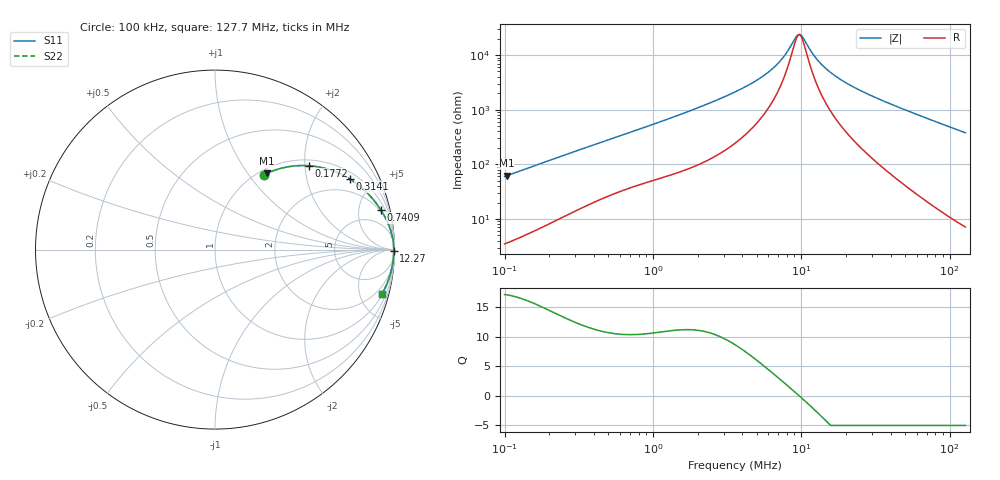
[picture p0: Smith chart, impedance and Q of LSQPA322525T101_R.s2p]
! LSQPA322525T101_R  S-PARAMETER MODEL  ( General Type )
! Model Generated by TAIYO YUDEN Corporation (http://www.ty-top.com)
! Version 2.0
! TAIYO YUDEN Control No. 100810NF25SB-FAC
! Copyright(c) 2007 TAIYO YUDEN CO.,LTD. All Rights Reserved.
! Product Description (link to TY-COMPAS)
! https://ds.yuden.co.jp/TYCOMPAS/or/detail?pn=LSQPA322525T101KR&u=M
! Products Name : Inductors
! Characteristics :
!  Inductance : 100 uH , SRF(min) : 6.0 MHz , DC Resistance(max) : 1.82 Ohm
!  Rated Current : Saturation :270 mA , Temp Rise : 340 mA (40 degC)
!  Case Size : 3.2 x 2.5 / 0.126 x 0.098 [mm/inch] , Thickness : 2.5 / 0.098 [mm/inch]
!  (Conditions: Temperature = 25 degC , DC Bias Current/Voltage = 0A / 0V)
! External Node Assignments :
!  1  o---GGG---o  2
! GND o---------o GND
! Frequency Range : 0.1MHz  -  127.746476MHz  [ 402 STEP ]
# MHz S RI R 50
! Freq[MHz].  S11 Real  S11 Imag  S21 Real  S21 Imag  S12 Real  S12 Imag  S22 Real  S22 Imag
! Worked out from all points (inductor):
!   401 points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, 100 kHz to 127.7 MHz, reference 50 ohm
!   read as one part in series: L = 94.6 uH near 103.6 kHz
!   highest Q = 17.1 at 103.6 kHz (marker M1), where L = 95 uH
!   self-resonance near 9.556 MHz
!   S11 on the Smith chart (normalised r, x): 100 kHz: 1.07, +1.19; 177.2 kHz: 1.14, +2.09; 314.1 kHz: 1.30, +3.61; 740.9 kHz: 1.78, +8.06; 12.27 MHz: open; 127.7 MHz: 1.14, -7.55
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0.1  0.2753 0.4184  0.7247 -0.4184  0.7247 -0.4184  0.2753 0.4184
0.103641  0.2887 0.4248  0.7113 -0.4248  0.7113 -0.4248  0.2887 0.4248
0.177218  0.5215 0.4674  0.4785 -0.4674  0.4785 -0.4674  0.5215 0.4674
0.314062  0.7495 0.3943  0.2505 -0.3943  0.2505 -0.3943  0.7495 0.3943
0.33137  0.7661 0.3835  0.2339 -0.3835  0.2339 -0.3835  0.7661 0.3835
0.740931  0.9235 0.2218  0.0765 -0.2218  0.0765 -0.2218  0.9235 0.2218
1.098062  0.9579 0.1595  0.0421 -0.1595  0.0421 -0.1595  0.9579 0.1595
2.127963  0.985 0.0844  0.015 -0.0844  0.015 -0.0844  0.985 0.0844
3.574164  0.9924 0.0464  0.00759 -0.0464  0.00759 -0.0464  0.9924 0.0464
5.020258  0.9945 0.0281  0.00552 -0.0281  0.00552 -0.0281  0.9945 0.0281
6.448345  0.9953 0.0167  0.00471 -0.0167  0.00471 -0.0167  0.9953 0.0167
7.574276  0.9956 0.00994  0.00441 -0.00994  0.00441 -0.00994  0.9956 0.00994
9.057322  0.9958 0.00269  0.00422 -0.00269  0.00422 -0.00269  0.9958 0.00269
9.556469  0.9958 0.000537  0.00419 -0.000537  0.00419 -0.000537  0.9958 0.000537
10.26505  0.9958 -0.00233  0.00417 0.00233  0.00417 0.00233  0.9958 -0.00233
11.84371  0.9958 -0.00811  0.00418 0.00811  0.00418 0.00811  0.9958 -0.00811
12.27495  0.9958 -0.00958  0.0042 0.00958  0.0042 0.00958  0.9958 -0.00958
14.67839  0.9956 -0.0171  0.00437 0.0171  0.00437 0.0171  0.9956 -0.0171
18.51973  0.9952 -0.0278  0.00483 0.0278  0.00483 0.0278  0.9952 -0.0278
25.55174  0.9939 -0.0452  0.00609 0.0452  0.00609 0.0452  0.9939 -0.0452
39.24654  0.9901 -0.0758  0.00988 0.0758  0.00988 0.0758  0.9901 -0.0758
127.7465  0.9304 -0.2453  0.0696 0.2453  0.0696 0.2453  0.9304 -0.2453
